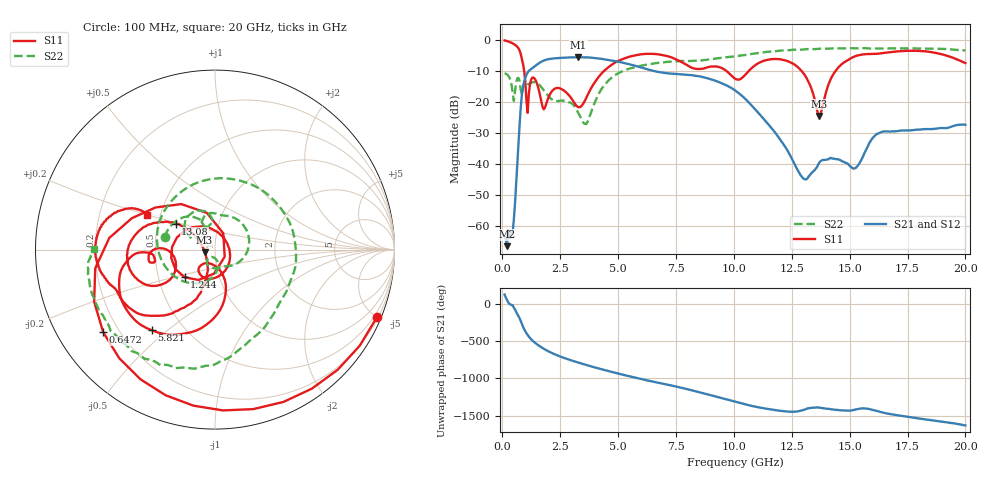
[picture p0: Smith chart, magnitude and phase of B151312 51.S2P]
!  2-Port S-parameters saved by WinCal
! VAR MeasName=S-Parameters (CALIBRATED_DATA) read from VNA (N5244A)
! VAR MeasDate=12/8/2015 5:47:47 PM
! VAR NAME=B151312 51
! VAR FILENAME=B151312 51.S2P
! VAR DATE=12/8/2015 5:47:47 PM
! VAR PHYS_PORTS=1,2
# Hz S DB R 50
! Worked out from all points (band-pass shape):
!   401 points, 100 MHz to 20 GHz, reference 50 ohm
!   highest |S21| = -5.59 dB at 3.284 GHz (marker M1); lowest = -66.4 dB at 199.5 MHz (marker M2)
!   |S21| within 3 dB of the highest: 1.388 GHz to 5.856 GHz (4.467 GHz wide, 123 % of centre)
!   lowest |S11| = -24.4 dB at 13.68 GHz (marker M3), VSWR 1.13, Z = 44.5 - j1.26 ohm
!   |S11| at or under -10 dB: 945.4 MHz to 4.394 GHz (3.449 GHz wide, 129 % of centre); 9.677 GHz to 10.65 GHz (969.4 MHz wide, 9.54 % of centre); 12.92 GHz to 14.39 GHz (1.469 GHz wide, 10.8 % of centre)
!   |S22| runs from -27.0 to -2.7 dB; largest |S21 - S12| = 0.0021
!   S11 on the Smith chart (normalised r, x): 100 MHz: 0.29, -4.99; 647.2 MHz: 0.14, -0.32; 1.244 GHz: 0.68, -0.22; 5.821 GHz: 0.33, -0.44; 13.08 GHz: 0.62, +0.19; 20 GHz: 0.42, +0.20
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1e8  -0.20 -22.6  -63.17 121.3  -63.38 127.2  -10.76 166.0
1.995e8  -0.38 -44.4  -66.35 51.6  -65.75 50.1  -11.11 150.8
4.4825e8  -1.13 -97.9  -61.86 -20.7  -62.42 -24.3  -17.07 114.2
6.4725e8  -2.22 -143.5  -39.96 -138.0  -39.89 -138.1  -12.36 132.5
8.96e8  -7.81 144.8  -15.11 50.4  -15.11 50.4  -15.37 116.0
1.24425e9  -12.80 -137.7  -9.38 -116.5  -9.38 -116.5  -13.79 65.0
1.5925e9  -16.57 119.4  -7.47 155.9  -7.47 155.9  -14.44 6.2
1.9905e9  -18.60 -52.7  -6.22 82.6  -6.22 82.7  -18.08 -46.2
2.5875e9  -15.97 -122.2  -5.78 3.4  -5.77 3.4  -19.55 -85.1
3.284e9  -21.67 -112.1  -5.59 -68.3  -5.59 -68.3  -23.51 -127.7
3.43325e9  -21.14 -93.5  -5.60 -82.3  -5.60 -82.3  -25.72 -127.2
4.478e9  -9.44 -85.1  -6.34 -173.0  -6.33 -172.9  -13.94 -112.6
5.82125e9  -4.87 -128.0  -8.52 84.2  -8.48 84.1  -8.61 123.1
6.7665e9  -4.70 -155.7  -10.35 20.6  -10.35 20.5  -7.40 42.3
8.259e9  -9.17 -175.4  -11.46 -84.1  -11.44 -84.3  -6.72 -31.0
1.005e10  -12.46 -173.4  -16.23 128.7  -16.22 128.6  -5.30 -69.3
1.308475e10  -11.60 146.6  -44.87 27.7  -44.89 27.1  -3.01 -114.6
1.338325e10  -16.41 144.3  -42.64 48.5  -42.64 48.3  -2.99 -117.6
1.368175e10  -24.45 -166.4  -39.60 50.3  -39.56 50.4  -2.85 -121.8
1.4627e10  -7.99 -121.3  -38.76 13.1  -38.79 12.9  -2.78 -132.2
1.67165e10  -4.02 -165.0  -29.49 -34.5  -29.40 -35.0  -2.73 -151.7
2e10  -7.47 152.8  -27.33 171.6  -27.45 171.2  -3.40 179.8
